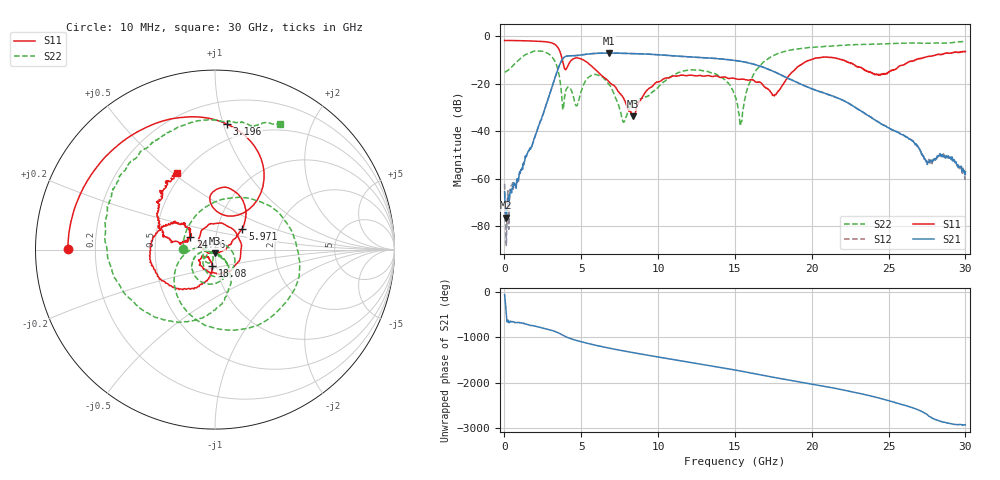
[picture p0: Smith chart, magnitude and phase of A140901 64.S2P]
!  2-Port S-parameters saved by WinCal
! VAR MeasName=S-Parameters (CALIBRATED_DATA) read from VNA (N5244A)
! VAR MeasDate=11/3/2014 9:37:05 AM
! VAR NAME=A140901 64
! VAR FILENAME=A140901 64.S2P
! VAR DATE=11/3/2014 9:37:05 AM
! VAR PHYS_PORTS=1,2
# Hz S RI R 50
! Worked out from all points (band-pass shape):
!   801 points, 10 MHz to 30 GHz, reference 50 ohm
!   highest |S21| = -7.06 dB at 6.795 GHz (marker M1); lowest = -76.5 dB at 122.5 MHz (marker M2)
!   |S21| within 3 dB of the highest: 3.734 GHz to 14.85 GHz (11.12 GHz wide, 120 % of centre)
!   lowest |S11| = -33.8 dB at 8.37 GHz (marker M3), VSWR 1.04, Z = 50.2 - j2.05 ohm
!   |S11| at or under -10 dB: 3.77 GHz to 4.371 GHz (600.9 MHz wide, 14.8 % of centre); 5.151 GHz to 19.89 GHz (14.74 GHz wide, 118 % of centre); 22.09 GHz to 26.73 GHz (4.637 GHz wide, 19 % of centre)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
!   |S22| runs from -37.8 to -2.1 dB; largest |S21 - S12| = 0.0025
!   S11 on the Smith chart (normalised r, x): 10 MHz: 0.10, +0.00; 3.196 GHz: 0.37, +1.03; 5.971 GHz: 1.32, +0.32; 18.08 GHz: 0.95, -0.17; 24.26 GHz: 0.75, +0.11; 30 GHz: 0.47, +0.52
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1e7  -0.8188 0.00203  0.000255 -0.000462  -0.000314 -0.000707  -0.1764 0.00418
1.224625e8  -0.8185 0.0397  -0.000113 -9.7e-05  3.39e-05 1.59e-05  -0.1736 0.0588
1.022162e9  -0.7428 0.3248  0.00108 0.000772  0.000916 0.000898  0.176 0.2884
1.884375e9  -0.5602 0.5651  0.00543 -0.00269  0.00545 -0.00269  0.4721 -0.0925
3.196438e9  0.0679 0.6989  -0.0857 -0.0658  -0.0852 -0.0658  -0.2115 -0.2555
3.833725e9  0.1581 0.2039  -0.168 0.3046  -0.1683 0.3039  -0.0161 -0.0244
5.033325e9  0.1368 0.2998  0.3737 -0.1604  0.374 -0.1601  0.075 0.0128
5.970512e9  0.1528 0.1175  -0.075 -0.4315  -0.0741 -0.4311  0.0299 -0.1539
6.795238e9  0.0987 0.0502  -0.4146 -0.1574  -0.4135 -0.1577  -0.0673 -0.0709
7.732425e9  0.0513 -0.00346  -0.3351 0.2823  -0.335 0.2817  -0.00278 -0.0152
8.369712e9  0.00192 -0.0204  -0.0809 0.4271  -0.0817 0.4261  0.0204 -0.0331
1.001916e10  -0.0902 0.0636  0.4085 0.0274  0.408 0.0268  0.056 -0.0635
1.155615e10  0.0369 0.1479  0.0504 -0.3737  0.0509 -0.3728  0.0208 -0.1803
1.305565e10  0.1432 -0.0265  -0.3435 -0.0851  -0.3423 -0.0855  -0.1128 -0.1468
1.5005e10  -0.0371 -0.1222  0.0624 0.303  0.0629 0.3032  -0.0544 -0.00782
1.537988e10  -0.0586 -0.1101  0.1707 0.2431  0.1713 0.2439  -0.00615 -0.0135
1.631706e10  -0.0816 -0.073  0.2524 -0.0247  0.2513 -0.025  0.0873 -0.1585
1.807898e10  -0.0151 -0.0894  -0.0695 -0.1313  -0.0685 -0.1316  -0.2324 -0.4024
2.002832e10  -0.269 -0.1875  -0.048 0.0611  -0.0487 0.061  -0.5738 -0.1155
2.426441e10  -0.1381 0.0711  -0.0158 -0.00342  -0.0158 -0.00364  -0.3661 0.5772
2.501416e10  -0.1651 0.0448  -0.00643 0.00979  -0.0065 0.00977  -0.2769 0.6448
3e10  -0.2108 0.4291  0.000911 -0.00107  0.000714 -0.00106  0.3611 0.6983
